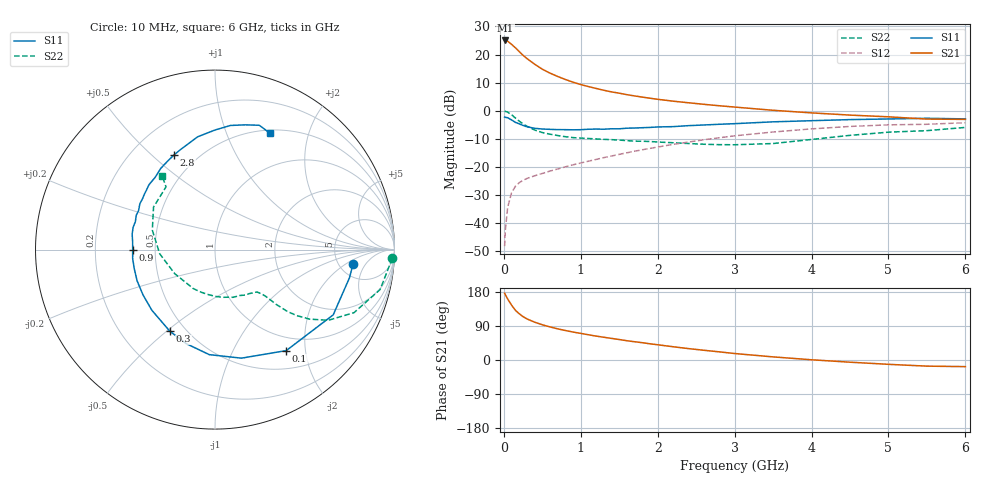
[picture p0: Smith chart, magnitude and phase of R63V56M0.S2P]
! SIEMENS Small Signal Semiconductors
! BFR193
! Si NPN RF Bipolar Junction Transistor in SOT23
! VCE = 3.5 V  IC = 6 mA
! Common Emitter S-Parameters:  May  1996
# GHz  S  MA  R  50
!  f  S11  S21  S12  S22
! GHz  MAG  ANG  MAG  ANG  MAG  ANG  MAG  ANG
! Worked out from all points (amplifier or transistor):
!   36 points, 10 MHz to 6 GHz, reference 50 ohm
!   highest |S21| = 25.0 dB at 20 MHz (marker M1)
!   |S21| within 3 dB of that: start of sweep to 164.5 MHz
!   unconditionally stable (mu >= 1): 853.8 MHz to 1.978 GHz
!   at 250 MHz: K = 0.48, MSG = 22.2 dB, |S12| = -24.7 dB
!   at 1.4 GHz: K = 1.06, MAG = 10.0 dB, |S12| = -16.1 dB
!   at 6 GHz: K = 0.96, MSG = 0.6 dB, |S12| = -4.2 dB
!   lowest NFmin = 1.20 dB at 450 MHz
!   S11 on the Smith chart (normalised r, x): 10 MHz: 6.69, -2.73; 100 MHz: 0.77, -1.65; 300 MHz: 0.41, -0.51; 900 MHz: 0.37, -0.00; 2.8 GHz: 0.37, +0.59; 6 GHz: 0.54, +1.44
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0.01  0.7734 -6.1  17.71 176.3  0.0039 89.5  0.9893 -2.8
0.02  0.7654 -11.9  17.84 172.0  0.0077 87.5  0.9749 -5.5
0.05  0.7523 -28.9  17.27 161.0  0.0192 76.2  0.9464 -13.6
0.1  0.6886 -54.8  15.25 145.0  0.0347 65.8  0.8504 -24.4
0.15  0.6226 -76.3  13.21 131.3  0.0453 57.9  0.7435 -32.0
0.2  0.5861 -93.1  11.31 122.0  0.0525 53.8  0.6541 -36.3
0.25  0.5482 -106.9  9.699 114.4  0.058 50.8  0.5856 -38.9
0.3  0.5199 -118.9  8.51 108.4  0.0624 49.8  0.5317 -40.5
0.4  0.4879 -136.1  6.755 99.9  0.0697 49.8  0.455 -41.9
0.5  0.4737 -148.0  5.494 93.0  0.0767 50.9  0.4097 -42.3
0.6  0.4676 -158.2  4.68 87.3  0.0846 52.0  0.3832 -42.7
0.7  0.4622 -166.8  4.081 82.2  0.0922 53.9  0.3627 -43.4
0.9  0.4586 -180.0  3.23 73.8  0.1094 56.5  0.3332 -45.2
1.1  0.4697 169.4  2.695 66.6  0.1269 58.3  0.3214 -48.6
1.3  0.4701 160.7  2.318 60.0  0.1469 59.2  0.3101 -52.4
1.6  0.4904 148.6  1.935 50.8  0.1789 59.4  0.2943 -60.1
2.2  0.5224 129.8  1.483 35.0  0.2523 56.3  0.27 -79.8
2.8  0.5755 113.2  1.229 21.5  0.331 49.7  0.2497 -107.9
3.5  0.636 98.7  1.021 8.2  0.4194 39.1  0.2614 -149.2
4.5  0.697 82.9  0.838 -5.8  0.5266 23.0  0.3655 162.8
5.5  0.7353 70.4  0.712 -16.2  0.5751 6.3  0.4433 128.0
6  0.7175 64.8  0.703 -17.5  0.6135 1.4  0.5057 125.6
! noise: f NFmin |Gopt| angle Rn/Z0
0.45  1.2  0.25  114  0.13
0.9  1.25  0.37  150  0.12
1.8  2  0.55  -158  0.12
